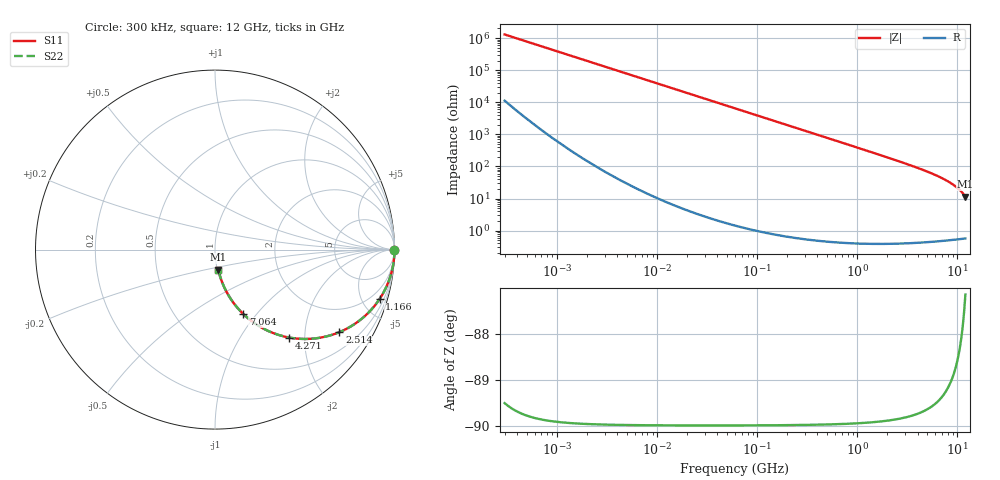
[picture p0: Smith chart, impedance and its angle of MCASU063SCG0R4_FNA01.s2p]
! MCASU063SCG0R4_FNA01  S-PARAMETER MODEL  ( Standard Model )
! Model Generated by TAIYO YUDEN Corporation (http://www.ty-top.com)
! Version 1.0
! TAIYO YUDEN Control No. 230609
! Copyright(c) 2023 TAIYO YUDEN CO.,LTD. All Rights Reserved.
! Product Description (link to TY-COMPAS)
! https://ds.yuden.co.jp/TYCOMPAS/or/detail?pn=MCASU063SCG0R4BFNA01&u=M
! Products Name : Multilayer Ceramic Capacitors
! Characteristics :
!  Capacitance : 0.4 [pF] , Rated Voltage : 50 [V] , TCC : CG / C0G
!  Case Size : 0.6 x 0.3 / 0.024 x 0.012 [mm/inch] , Thickness : 0.3 / 0.012 [mm/inch]
!  (Conditions: Temperature = 25 [degC] , DC Bias Voltage = 0 [V])
! External Node Assignments :
!  1  o---| |---o  2
! GND o---------o GND
! Frequency Range : 0.3MHz  -  12000MHz  [ 401 STEP ]
# MHZ S RI R 50
! Freq[MHz].  S11 Real  S11 Imag  S21 Real  S21 Imag  S12 Real  S12 Imag  S22 Real  S22 Imag
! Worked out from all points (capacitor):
!   401 points, 300 kHz to 12 GHz, reference 50 ohm
!   read as one part in series: C = 408 fF near 316.3 kHz
!   lowest |Z| = 11.5 ohm at 12 GHz (marker M1)
!   S11 on the Smith chart (normalised r, x): 300 kHz: open; 1.166 GHz: 1.01, -6.64; 2.514 GHz: 1.01, -3.01; 4.271 GHz: 1.01, -1.68; 7.064 GHz: 1.01, -0.86; 12 GHz: 1.01, -0.23
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0.3  1 -7.7e-05  6.72e-07 7.7e-05  6.72e-07 7.7e-05  1 -7.7e-05
0.370819  1 -9.51e-05  5.94e-07 9.51e-05  5.94e-07 9.51e-05  1 -9.51e-05
0.412271  1 -0.000106  5.64e-07 0.000106  5.64e-07 0.000106  1 -0.000106
1.769972  1 -0.000454  5.91e-07 0.000454  5.91e-07 0.000454  1 -0.000454
10.44266  1 -0.00268  7.88e-06 0.00268  7.88e-06 0.00268  1 -0.00268
60  0.9998 -0.0154  0.00024 0.0154  0.00024 0.0154  0.9998 -0.0154
164.1901  0.9982 -0.0421  0.00179 0.0421  0.00179 0.0421  0.9982 -0.0421
353.9943  0.9918 -0.0901  0.00823 0.0901  0.00823 0.0901  0.9918 -0.0901
651.0506  0.9726 -0.1628  0.0274 0.1628  0.0274 0.1628  0.9726 -0.1628
1166.079  0.9166 -0.2759  0.0834 0.2759  0.0834 0.2759  0.9166 -0.2759
1560.575  0.8588 -0.3475  0.1412 0.3475  0.1412 0.3475  0.8588 -0.3475
2088.533  0.7695 -0.4201  0.2305 0.4201  0.2305 0.4201  0.7695 -0.4201
2514.07  0.6936 -0.4597  0.3064 0.4597  0.3064 0.4597  0.6936 -0.4597
3364.605  0.5471 -0.4959  0.4529 0.4959  0.4529 0.4959  0.5471 -0.4959
4270.516  0.4129 -0.4898  0.5871 0.4898  0.5871 0.4898  0.4129 -0.4898
5420.343  0.2818 -0.4463  0.7182 0.4463  0.7182 0.4463  0.2818 -0.4463
7064.448  0.1576 -0.3589  0.8424 0.3589  0.8424 0.3589  0.1576 -0.3589
8281.503  0.0996 -0.2918  0.9004 0.2918  0.9004 0.2918  0.0996 -0.2918
9454.42  0.0618 -0.2304  0.9382 0.2304  0.9382 0.2304  0.0618 -0.2304
10511.28  0.0387 -0.1788  0.9613 0.1788  0.9613 0.1788  0.0387 -0.1788
11380.75  0.0254 -0.1391  0.9746 0.1391  0.9746 0.1391  0.0254 -0.1391
12000  0.0185 -0.1122  0.9815 0.1122  0.9815 0.1122  0.0185 -0.1122
